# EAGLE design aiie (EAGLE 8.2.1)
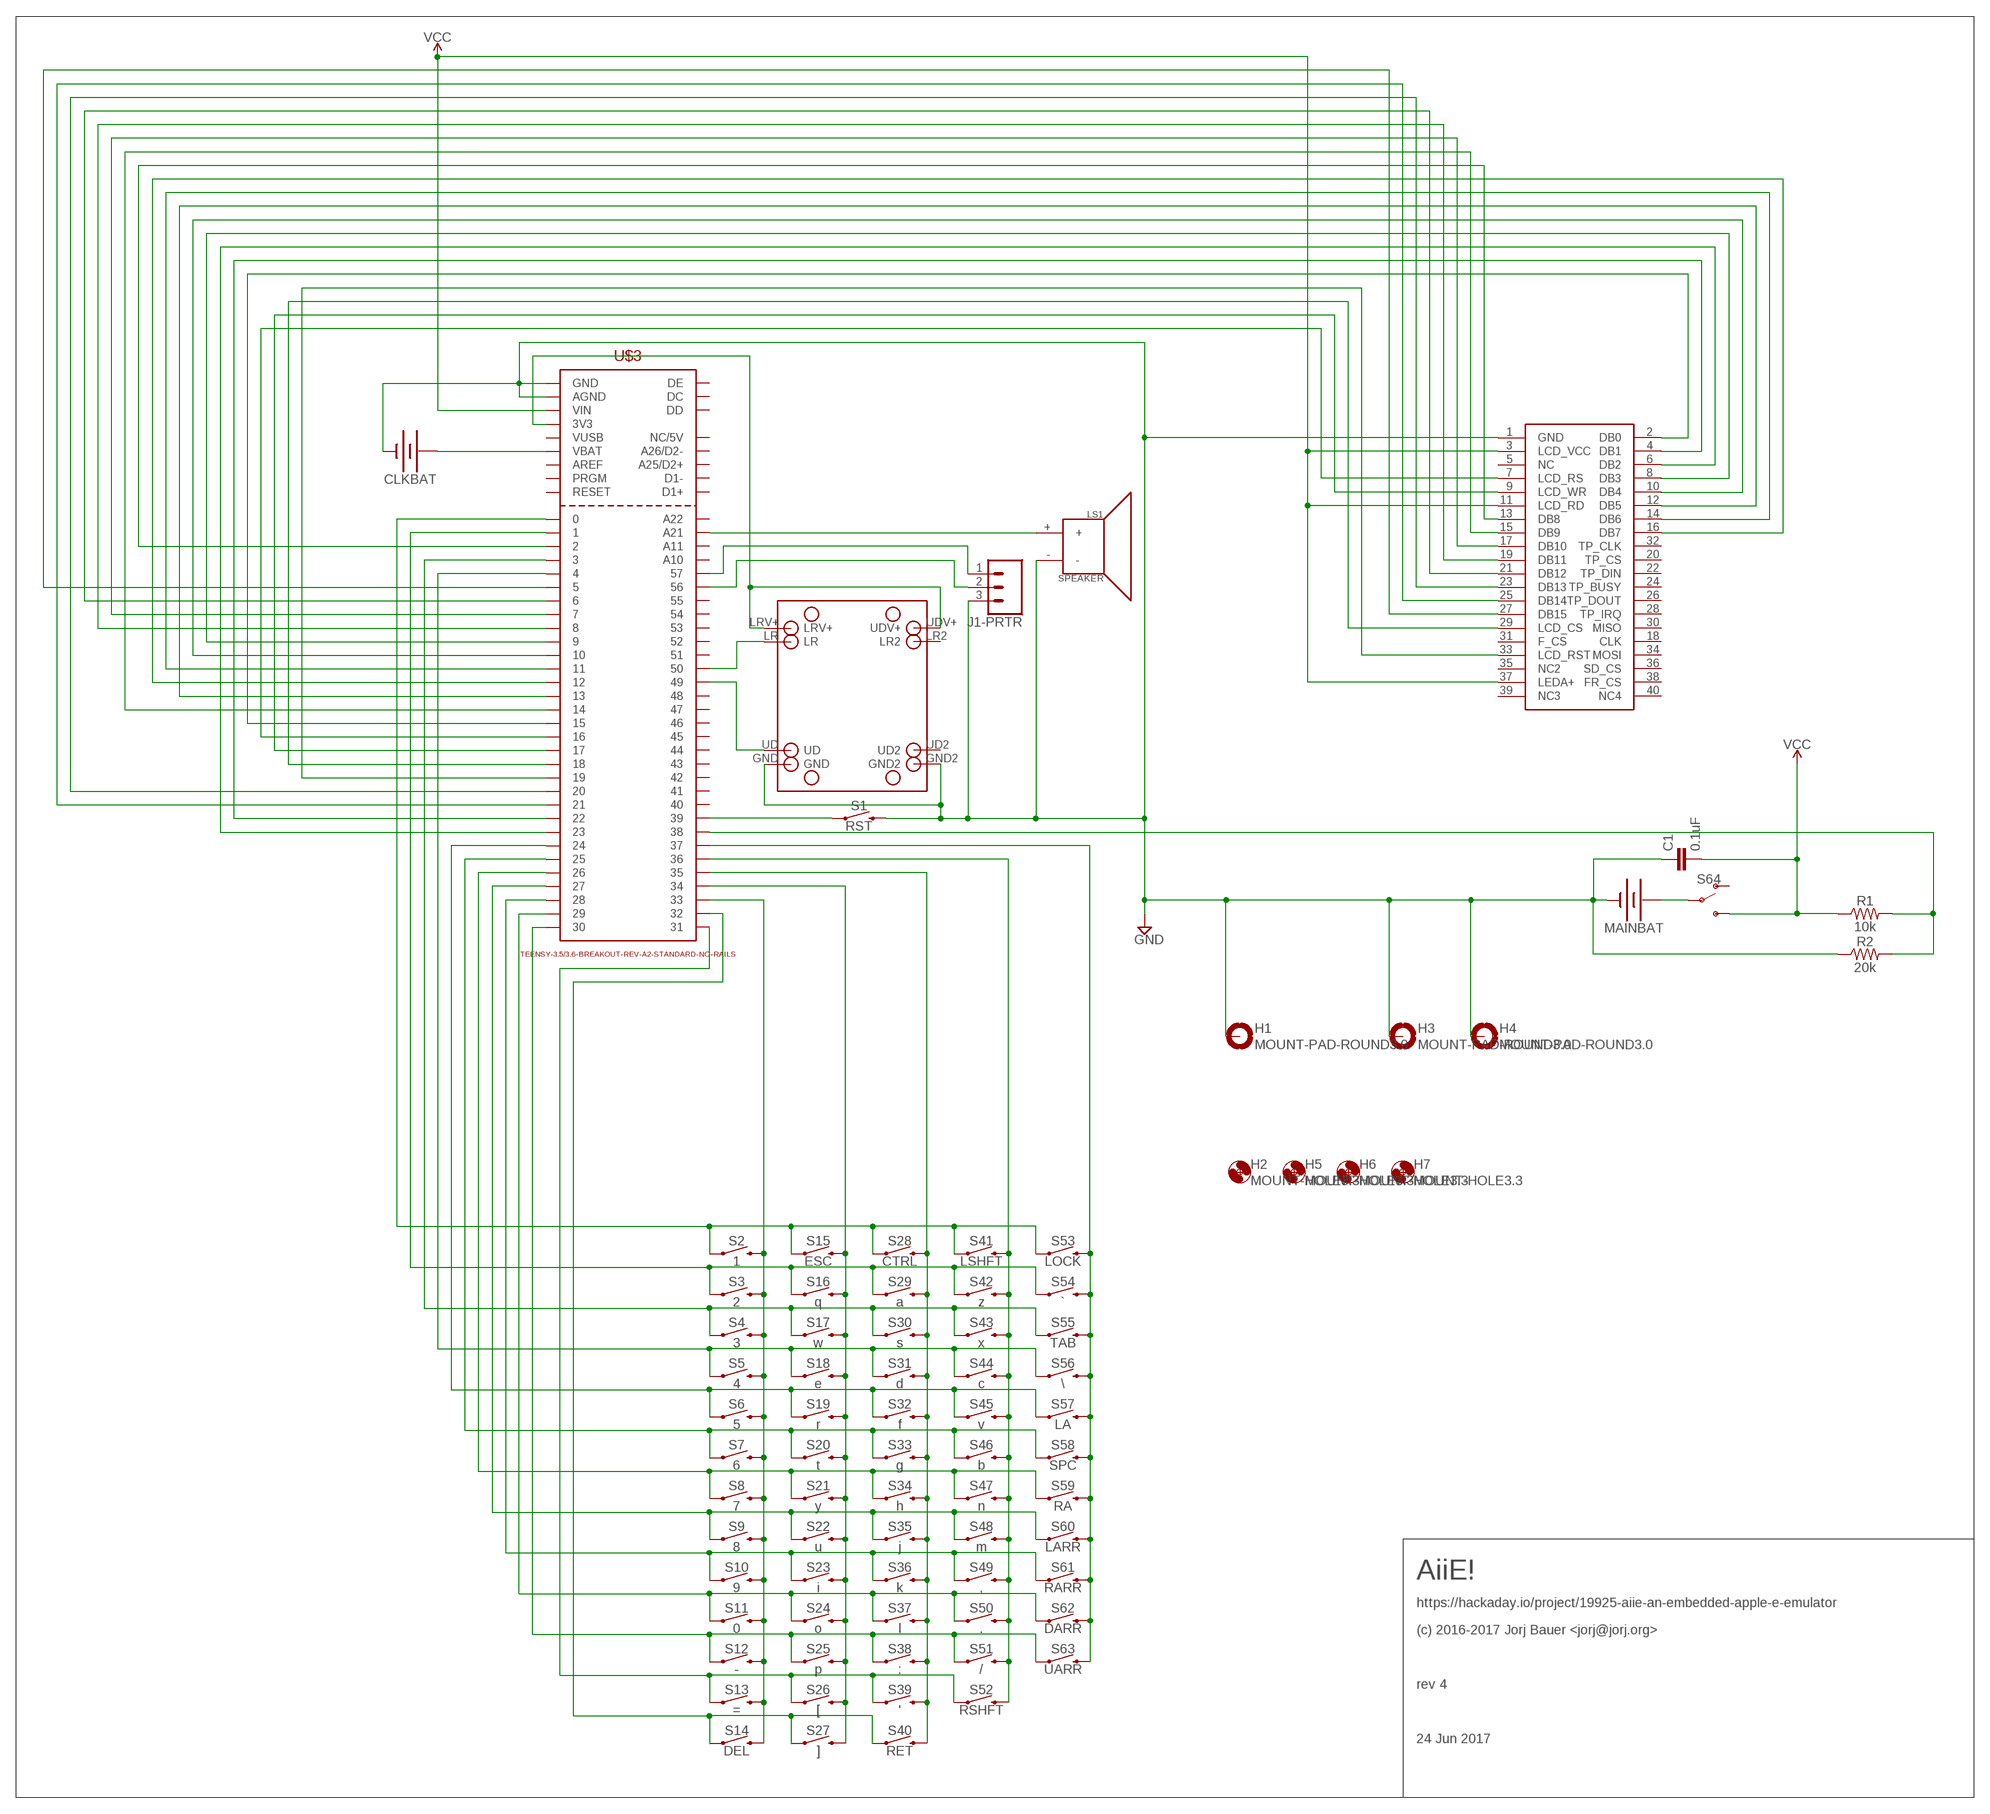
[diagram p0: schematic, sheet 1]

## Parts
C1  0.1uF  C-EU025_050-025X075  [C025_050-025X075]
CLKBAT  BATTERY-20MM_PTH  [BATTCOM_20MM_PTH]
H1  MOUNT-PAD-ROUND3.0  [3,0-PAD]
H2  MOUNT-HOLE3.3  [3,3]
H3  MOUNT-PAD-ROUND3.0  [3,0-PAD]
H4  MOUNT-PAD-ROUND3.0  [3,0-PAD]
H5  MOUNT-HOLE3.3  [3,3]
H6  MOUNT-HOLE3.3  [3,3]
H7  MOUNT-HOLE3.3  [3,3]
J1-PRTR  CONN_03  [1X03]
LS1  SPEAKER  [PCB_MOUNT_SPEAKER]
MAINBAT  BATTERY-18650  [BATTERY_18650-HOLDER]
R1  10k  10KOHM-HORIZ-1/4W-1%  [AXIAL-0.3]
R2  20k  10KOHM-HORIZ-1/4W-1%  [AXIAL-0.3]
S1  RST  MOMENTARY-SWITCH-SPST-PTH-6.0MM  [TACTILE_SWITCH_PTH_6.0MM]
S2  1  MOMENTARY-SWITCH-SPST-PTH-6.0MM  [TACTILE_SWITCH_PTH_6.0MM]
S3  2  MOMENTARY-SWITCH-SPST-PTH-6.0MM  [TACTILE_SWITCH_PTH_6.0MM]
S4  3  MOMENTARY-SWITCH-SPST-PTH-6.0MM  [TACTILE_SWITCH_PTH_6.0MM]
S5  4  MOMENTARY-SWITCH-SPST-PTH-6.0MM  [TACTILE_SWITCH_PTH_6.0MM]
S6  5  MOMENTARY-SWITCH-SPST-PTH-6.0MM  [TACTILE_SWITCH_PTH_6.0MM]
S7  6  MOMENTARY-SWITCH-SPST-PTH-6.0MM  [TACTILE_SWITCH_PTH_6.0MM]
S8  7  MOMENTARY-SWITCH-SPST-PTH-6.0MM  [TACTILE_SWITCH_PTH_6.0MM]
S9  8  MOMENTARY-SWITCH-SPST-PTH-6.0MM  [TACTILE_SWITCH_PTH_6.0MM]
S10  9  MOMENTARY-SWITCH-SPST-PTH-6.0MM  [TACTILE_SWITCH_PTH_6.0MM]
S11  0  MOMENTARY-SWITCH-SPST-PTH-6.0MM  [TACTILE_SWITCH_PTH_6.0MM]
S12  -  MOMENTARY-SWITCH-SPST-PTH-6.0MM  [TACTILE_SWITCH_PTH_6.0MM]
S13  =  MOMENTARY-SWITCH-SPST-PTH-6.0MM  [TACTILE_SWITCH_PTH_6.0MM]
S14  DEL  MOMENTARY-SWITCH-SPST-PTH-6.0MM  [TACTILE_SWITCH_PTH_6.0MM]
S15  ESC  MOMENTARY-SWITCH-SPST-PTH-6.0MM  [TACTILE_SWITCH_PTH_6.0MM]
S16  q  MOMENTARY-SWITCH-SPST-PTH-6.0MM  [TACTILE_SWITCH_PTH_6.0MM]
S17  w  MOMENTARY-SWITCH-SPST-PTH-6.0MM  [TACTILE_SWITCH_PTH_6.0MM]
S18  e  MOMENTARY-SWITCH-SPST-PTH-6.0MM  [TACTILE_SWITCH_PTH_6.0MM]
S19  r  MOMENTARY-SWITCH-SPST-PTH-6.0MM  [TACTILE_SWITCH_PTH_6.0MM]
S20  t  MOMENTARY-SWITCH-SPST-PTH-6.0MM  [TACTILE_SWITCH_PTH_6.0MM]
S21  y  MOMENTARY-SWITCH-SPST-PTH-6.0MM  [TACTILE_SWITCH_PTH_6.0MM]
S22  u  MOMENTARY-SWITCH-SPST-PTH-6.0MM  [TACTILE_SWITCH_PTH_6.0MM]
S23  i  MOMENTARY-SWITCH-SPST-PTH-6.0MM  [TACTILE_SWITCH_PTH_6.0MM]
S24  o  MOMENTARY-SWITCH-SPST-PTH-6.0MM  [TACTILE_SWITCH_PTH_6.0MM]
S25  p  MOMENTARY-SWITCH-SPST-PTH-6.0MM  [TACTILE_SWITCH_PTH_6.0MM]
S26  [  MOMENTARY-SWITCH-SPST-PTH-6.0MM  [TACTILE_SWITCH_PTH_6.0MM]
S27  ]  MOMENTARY-SWITCH-SPST-PTH-6.0MM  [TACTILE_SWITCH_PTH_6.0MM]
S28  CTRL  MOMENTARY-SWITCH-SPST-PTH-6.0MM  [TACTILE_SWITCH_PTH_6.0MM]
S29  a  MOMENTARY-SWITCH-SPST-PTH-6.0MM  [TACTILE_SWITCH_PTH_6.0MM]
S30  s  MOMENTARY-SWITCH-SPST-PTH-6.0MM  [TACTILE_SWITCH_PTH_6.0MM]
S31  d  MOMENTARY-SWITCH-SPST-PTH-6.0MM  [TACTILE_SWITCH_PTH_6.0MM]
S32  f  MOMENTARY-SWITCH-SPST-PTH-6.0MM  [TACTILE_SWITCH_PTH_6.0MM]
S33  g  MOMENTARY-SWITCH-SPST-PTH-6.0MM  [TACTILE_SWITCH_PTH_6.0MM]
S34  h  MOMENTARY-SWITCH-SPST-PTH-6.0MM  [TACTILE_SWITCH_PTH_6.0MM]
S35  j  MOMENTARY-SWITCH-SPST-PTH-6.0MM  [TACTILE_SWITCH_PTH_6.0MM]
S36  k  MOMENTARY-SWITCH-SPST-PTH-6.0MM  [TACTILE_SWITCH_PTH_6.0MM]
S37  l  MOMENTARY-SWITCH-SPST-PTH-6.0MM  [TACTILE_SWITCH_PTH_6.0MM]
S38  ;  MOMENTARY-SWITCH-SPST-PTH-6.0MM  [TACTILE_SWITCH_PTH_6.0MM]
S39  '  MOMENTARY-SWITCH-SPST-PTH-6.0MM  [TACTILE_SWITCH_PTH_6.0MM]
S40  RET  MOMENTARY-SWITCH-SPST-PTH-6.0MM  [TACTILE_SWITCH_PTH_6.0MM]
S41  LSHFT  MOMENTARY-SWITCH-SPST-PTH-6.0MM  [TACTILE_SWITCH_PTH_6.0MM]
S42  z  MOMENTARY-SWITCH-SPST-PTH-6.0MM  [TACTILE_SWITCH_PTH_6.0MM]
S43  x  MOMENTARY-SWITCH-SPST-PTH-6.0MM  [TACTILE_SWITCH_PTH_6.0MM]
S44  c  MOMENTARY-SWITCH-SPST-PTH-6.0MM  [TACTILE_SWITCH_PTH_6.0MM]
S45  v  MOMENTARY-SWITCH-SPST-PTH-6.0MM  [TACTILE_SWITCH_PTH_6.0MM]
S46  b  MOMENTARY-SWITCH-SPST-PTH-6.0MM  [TACTILE_SWITCH_PTH_6.0MM]
S47  n  MOMENTARY-SWITCH-SPST-PTH-6.0MM  [TACTILE_SWITCH_PTH_6.0MM]
S48  m  MOMENTARY-SWITCH-SPST-PTH-6.0MM  [TACTILE_SWITCH_PTH_6.0MM]
S49  ,  MOMENTARY-SWITCH-SPST-PTH-6.0MM  [TACTILE_SWITCH_PTH_6.0MM]
S50  .  MOMENTARY-SWITCH-SPST-PTH-6.0MM  [TACTILE_SWITCH_PTH_6.0MM]
S51  /  MOMENTARY-SWITCH-SPST-PTH-6.0MM  [TACTILE_SWITCH_PTH_6.0MM]
S52  RSHFT  MOMENTARY-SWITCH-SPST-PTH-6.0MM  [TACTILE_SWITCH_PTH_6.0MM]
S53  LOCK  MOMENTARY-SWITCH-SPST-PTH-6.0MM  [TACTILE_SWITCH_PTH_6.0MM]
S54  `  MOMENTARY-SWITCH-SPST-PTH-6.0MM  [TACTILE_SWITCH_PTH_6.0MM]
S55  TAB  MOMENTARY-SWITCH-SPST-PTH-6.0MM  [TACTILE_SWITCH_PTH_6.0MM]
S56  \\  MOMENTARY-SWITCH-SPST-PTH-6.0MM  [TACTILE_SWITCH_PTH_6.0MM]
S57  LA  MOMENTARY-SWITCH-SPST-PTH-6.0MM  [TACTILE_SWITCH_PTH_6.0MM]
S58  SPC  MOMENTARY-SWITCH-SPST-PTH-6.0MM  [TACTILE_SWITCH_PTH_6.0MM]
S59  RA  MOMENTARY-SWITCH-SPST-PTH-6.0MM  [TACTILE_SWITCH_PTH_6.0MM]
S60  LARR  MOMENTARY-SWITCH-SPST-PTH-6.0MM  [TACTILE_SWITCH_PTH_6.0MM]
S61  RARR  MOMENTARY-SWITCH-SPST-PTH-6.0MM  [TACTILE_SWITCH_PTH_6.0MM]
S62  DARR  MOMENTARY-SWITCH-SPST-PTH-6.0MM  [TACTILE_SWITCH_PTH_6.0MM]
S63  UARR  MOMENTARY-SWITCH-SPST-PTH-6.0MM  [TACTILE_SWITCH_PTH_6.0MM]
S64  SWITCH-SPDT-PTH-11.6X4.0MM  [SWITCH_SPDT_PTH_11.6X4.0MM]
U$1  PARALLAX2AXIS  [PARALLAX2AXIS]
U$2  SAINSMART32LCDRAW  [2X20]
U$3  TEENSY-3.5/3.6-BREAKOUT-REV-A2-STANDARD-NO-RAILS  [TEENSY-3.5/3.6-BREAKOUT-REV-A2-STANDARD-NO-RAILS]

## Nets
GND [ground]: C1.1 CLKBAT.2(-) H1.B3,0(MOUNT) H3.B3,0(MOUNT) H4.B3,0(MOUNT) J1-PRTR.3 LS1.- MAINBAT.GND@1(-) R2.P$1 S1.3 U$1.GND U$1.GND2 U$2.1(GND) U$3.AGND U$3.GND@1(GND) U$3.GND@2(GND)
N$1: S1.1 U$3.39
N$2: S2.3 S3.3 S4.3 S5.3 S6.3 S7.3 S8.3 S9.3 S10.3 S11.3 S12.3 S13.3 S14.3 U$3.33
N$3: S15.3 S16.3 S17.3 S18.3 S19.3 S20.3 S21.3 S22.3 S23.3 S24.3 S25.3 S26.3 S27.3 U$3.34
N$4: S28.3 S29.3 S30.3 S31.3 S32.3 S33.3 S34.3 S35.3 S36.3 S37.3 S38.3 S39.3 S40.3 U$3.35
N$5: S41.3 S42.3 S43.3 S44.3 S45.3 S46.3 S47.3 S48.3 S49.3 S50.3 S51.3 S52.3 U$3.36
N$6: S53.3 S54.3 S55.3 S56.3 S57.3 S58.3 S59.3 S60.3 S61.3 S62.3 S63.3 U$3.37
N$7: S2.1 S15.1 S28.1 S41.1 S53.1 U$3.0
N$8: S4.1 S17.1 S30.1 S43.1 S55.1 U$3.3
N$9: S3.1 S16.1 S29.1 S42.1 S54.1 U$3.1
N$10: U$2.7(LCD_RS) U$3.16
N$11: S5.1 S18.1 S31.1 S44.1 S56.1 U$3.4
N$12: U$2.9(LCD_WR) U$3.17
N$13: S6.1 S19.1 S32.1 S45.1 S57.1 U$3.24
N$14: U$2.29(LCD_CS) U$3.18
N$15: S7.1 S20.1 S33.1 S46.1 S58.1 U$3.25
N$16: U$2.33(LCD_RST) U$3.19
N$17: S8.1 S21.1 S34.1 S47.1 S59.1 U$3.26
N$18: U$2.2(DB0) U$3.15
N$19: S9.1 S22.1 S35.1 S48.1 S60.1 U$3.27
N$20: U$2.4(DB1) U$3.22
N$21: S10.1 S23.1 S36.1 S49.1 S61.1 U$3.28
N$22: U$2.6(DB2) U$3.23
N$23: S11.1 S24.1 S37.1 S50.1 S62.1 U$3.29
N$24: U$2.8(DB3) U$3.9
N$25: S12.1 S25.1 S38.1 S51.1 S63.1 U$3.30
N$26: S13.1 S26.1 S39.1 S52.1 U$3.31
N$27: S14.1 S27.1 S40.1 U$3.32
N$28: U$2.10(DB4) U$3.10
N$29: U$2.12(DB5) U$3.13
N$30: U$2.14(DB6) U$3.11
N$31: U$2.16(DB7) U$3.12
N$32: U$2.13(DB8) U$3.2
N$33: U$2.15(DB9) U$3.14
N$34: U$2.17(DB10) U$3.7
N$35: U$2.19(DB11) U$3.8
N$36: U$2.21(DB12) U$3.6
N$37: U$2.23(DB13) U$3.20
N$38: U$2.25(DB14) U$3.21
N$39: U$2.27(DB15) U$3.5
N$40 [vcc]: MAINBAT.PWR@1(+) S64.2(P)
N$41: LS1.+ U$3.A21
N$42: U$1.LR U$3.50
N$43: J1-PRTR.2 U$3.56
N$44: R1.P$2 R2.P$2 U$3.38
N$45: J1-PRTR.1 U$3.57
N$46: U$1.UD U$3.49
N$47: U$1.LRV+ U$1.UDV+ U$3.3V3
N$48: CLKBAT.1(+) U$3.VBAT
VCC [vcc]: C1.2 R1.P$1 S64.3(S) U$2.3(LCD_VCC) U$2.11(LCD_RD) U$2.37(LEDA+) U$3.VIN
Unconnected: S64.1(O) U$1.LR2 U$1.UD2 U$2.5(NC) U$2.18(CLK) U$2.20(TP_CS) U$2.22(TP_DIN) U$2.24(TP_BUSY) U$2.26(TP_DOUT) U$2.28(TP_IRQ) U$2.30(MISO) U$2.31(F_CS) U$2.32(TP_CLK) U$2.34(MOSI) U$2.35(NC2) U$2.36(SD_CS) U$2.38(FR_CS) U$2.39(NC3) U$2.40(NC4) U$3.40 U$3.41 U$3.42 U$3.43 U$3.44 U$3.45 U$3.46 U$3.47 U$3.48 U$3.51 U$3.52 U$3.53 U$3.54 U$3.55 U$3.A10 U$3.A11 U$3.A22 U$3.A25/D2+ U$3.A26/D2- U$3.AREF U$3.D1+ U$3.D1- U$3.DC U$3.DD U$3.DE U$3.NC/V5(NC/5V) U$3.PRGM U$3.RESET U$3.VUSB

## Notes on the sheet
- AiiE!
- https://hackaday.io/project/19925-aiie-an-embedded-apple-e-emulator
- (c) 2016-2017 Jorj Bauer <jorj@jorj.org>
- rev 4
- 24 Jun 2017

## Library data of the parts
C1 = rcl:C-EU: CAPACITOR, European symbol
CLKBAT = SparkFun-Batteries:BATTERY: Battery - Single Cell; PROD_ID: BATT-09031; SF_SKU: PRT-00783
H1 H3 H4 = holes:MOUNT-PAD-ROUND: MOUNTING PAD, round
H2 H5-H7 = holes:MOUNT-HOLE: MOUNTING HOLE with drill center marker
J1-PRTR = SparkFun-Connectors:CONN_03: Multi connection point. Often used as Generic Header-pin footprint for 0.1 inch spaced/style header connections On any of the 0.1 inch spaced packages, you can populate with these: Break Away Headers - Straight (PRT-00116) Break Away Male Headers - Right Angle (PRT-00553) Female Headers (PRT-00115)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
LS1 = SparkFun-Electromechanical:SPEAKER: Speaker; PROD_ID: COMP-11789; SF_SKU: COM-11089
MAINBAT = SparkFun-Batteries:BATTERY: Battery - Single Cell; PROD_ID: BATT-12327; SF_SKU: PRT-13113
R1 = SparkFun-Resistors:10KOHM: 10kΩ resistor; PROD_ID: RES-12183
R2 = SparkFun-Resistors:10KOHM: 10kΩ resistor; PROD_ID: RES-12183; VALUE: 10k
S1-S63 = SparkFun-Switches:MOMENTARY-SWITCH-SPST: Momentary Switch (Pushbutton) - SPST; PROD_ID: SWCH-08441; SF_SKU: COM-00097
S64 = SparkFun-Switches:SWITCH-SPDT: Single Pole, Double Throw (SPDT) Switch Single-pole, double-throw (SPDT) switch. Variant Overview SMD-AYZ0202 Surface Mount DPDT Switch (COM-00597) Used on e.g. LilyPad Arduino USB - ATmega32U4 Board PTH-11.6X4.0MM SPDT Mini Power Switch (COM-00102) Used on e.g. SparkFun Simon Says - Through-Hole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; PROD_ID: SWCH-08261; SF_SKU: COM-00102
U$1 = jorjlib:PARALLAX2AXIS
U$2 = jorjlib:SAINSMART32LCD
U$3 = Teensy-Breakout-Eagle-Library:TEENSY-3.5/3.6-BREAKOUT-REV-A2-STANDARD

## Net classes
0 default: width 0.254 mm, clearance 0.203 mm
1 ground: width 0.356 mm, clearance 0.203 mm
2 vcc: width 0.356 mm, clearance 0.203 mm

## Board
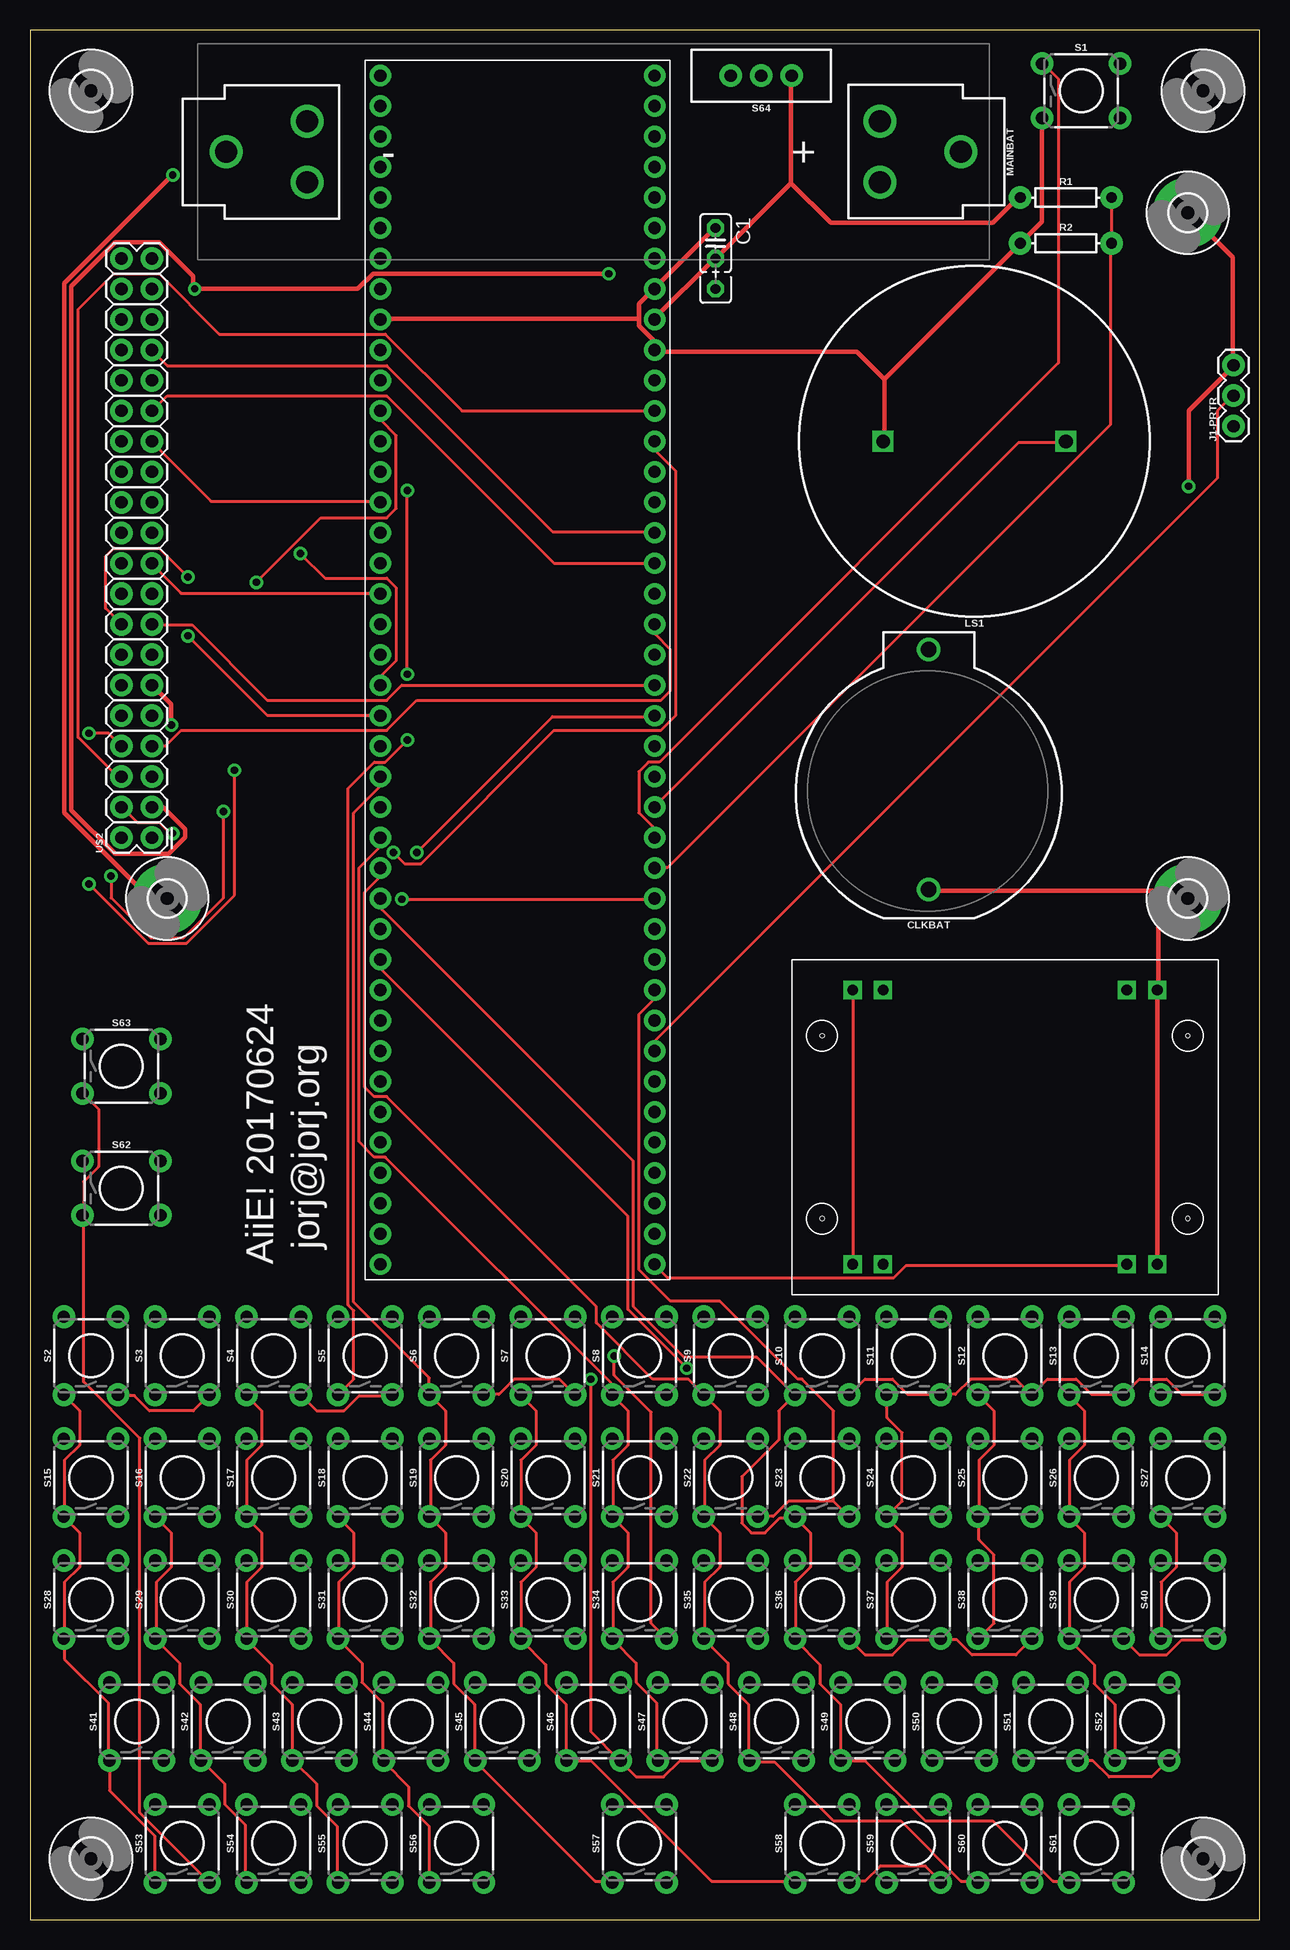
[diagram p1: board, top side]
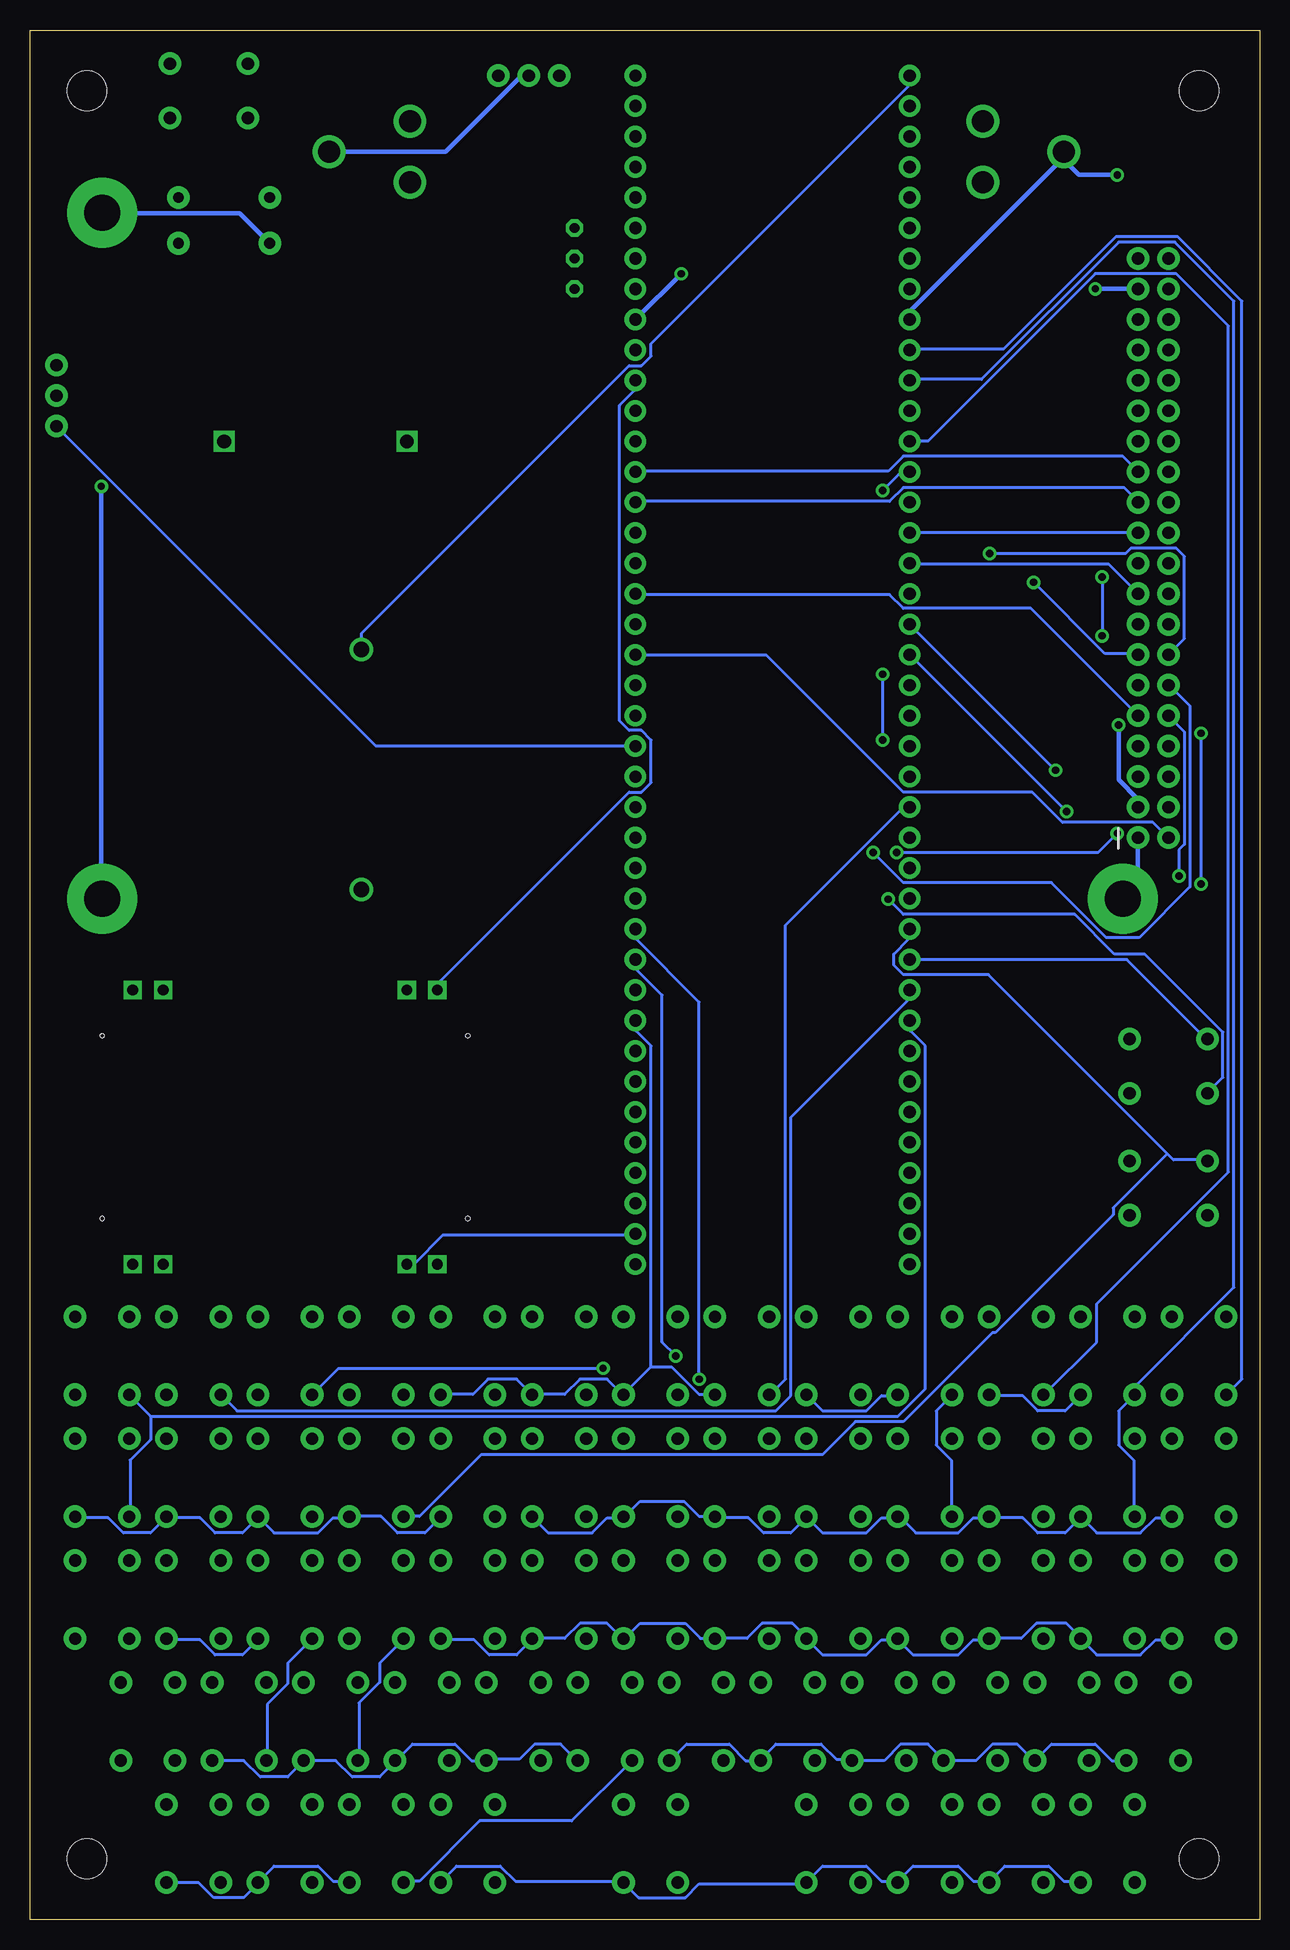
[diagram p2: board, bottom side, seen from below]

Size 102.54 x 157.47 mm. Coordinates in mm from the lower left corner, seen from the top.
Outline: 0,0 102.54,0 102.54,157.47 0,157.47 0,0
Copper layers (1*16): Top 0.035mm / dielectric 1.5mm / Bottom 0.035mm
Design rules "default *": minimum track width 10mil, minimum drill 24mil, track to track 8mil, track to pad 8mil, pad to pad 8mil, via to via 8mil, smd to smd 8mil, copper to edge 40mil, drill to drill 8mil, minimum pad ring 12mil, minimum via ring 10mil, stop-mask expansion 4mil, vias tented up to drill 0mil, thermal gap 10mil

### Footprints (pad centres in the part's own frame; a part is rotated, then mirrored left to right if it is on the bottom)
C025_050-025X075 = drill 0.813 octagon: 1 -1.27,0; 2 1.27,0; 3 3.81,0
BATTCOM_20MM_PTH = drill 1.3: 1 11.85,0; 2 -8.15,0
3,0-PAD = drill 3 pad 5.842: B3,0 0,0
3,3 = hole 3.3: 0,0
1X03 = drill 1.016 pad 1.88: 1 0,0; 2 2.54,0; 3 5.08,0
PCB_MOUNT_SPEAKER = drill 1.143 square: + -7.62,0; - 7.62,0
BATTERY_18650-HOLDER = drill 1.829: GND@1 30.628,0.01; GND@2 23.88,2.55; GND@3 23.88,-2.53; PWR@1 -30.628,-0.01; PWR@2 -23.88,2.53; PWR@3 -23.88,-2.55
AXIAL-0.3 = drill 0.9 pad 1.88: P$1 -3.81,0; P$2 3.81,0
TACTILE_SWITCH_PTH_6.0MM = drill 1.016 pad 1.88: 1 -3.251,2.261; 2 3.251,2.261; 3 -3.251,-2.261; 4 3.251,-2.261
SWITCH_SPDT_PTH_11.6X4.0MM = drill 1.016 pad 1.88: 1 0,2.54; 2 0,0; 3 0,-2.54
PARALLAX2AXIS = drill 0.9 square: GND 2.54,5.08; GND2 25.4,5.08; LR 2.54,27.94; LR2 25.4,27.94; LRV+ 2.54,30.48; UD 2.54,7.62; UD2 25.4,7.62; UDV+ 25.4,30.48 | hole 0.35: 21.59,33.02; 6.35,33.02; 6.35,2.54; 21.59,2.54
2X20 = drill 1.016 pad 1.88: 1 0,0; 2 0,2.54; 3 2.54,0; 4 2.54,2.54; 5 5.08,0; 6 5.08,2.54; 7 7.62,0; 8 7.62,2.54; 9 10.16,0; 10 10.16,2.54; 11 12.7,0; 12 12.7,2.54; 13 15.24,0; 14 15.24,2.54; 15 17.78,0; 16 17.78,2.54; 17 20.32,0; 18 20.32,2.54; 19 22.86,0; 20 22.86,2.54; 21 25.4,0; 22 25.4,2.54; 23 27.94,0; 24 27.94,2.54; 25 30.48,0; 26 30.48,2.54; 27 33.02,0; 28 33.02,2.54; 29 35.56,0; 30 35.56,2.54; 31 38.1,0; 32 38.1,2.54; 33 40.64,0; 34 40.64,2.54; 35 43.18,0; 36 43.18,2.54; 37 45.72,0; 38 45.72,2.54; 39 48.26,0; 40 48.26,2.54
TEENSY-3.5/3.6-BREAKOUT-REV-A2-STANDARD-NO-RAILS = drill 1.016 pad 1.778: 0 24.13,1.27; 1 26.67,1.27; 2 29.21,1.27; 3 31.75,1.27; 3V3 26.67,24.13; 4 34.29,1.27; 5 36.83,1.27; 6 39.37,1.27; 7 41.91,1.27; 8 44.45,1.27; 9 46.99,1.27; 10 49.53,1.27; 11 52.07,1.27; 12 54.61,1.27; 13 54.61,24.13; 14 52.07,24.13; 15 49.53,24.13; 16 46.99,24.13; 17 44.45,24.13; 18 41.91,24.13; 19 39.37,24.13; 20 36.83,24.13; 21 34.29,24.13; 22 31.75,24.13; 23 29.21,24.13; 24 59.69,1.27; 25 62.23,1.27; 26 64.77,1.27; 27 67.31,1.27; 28 69.85,1.27; 29 72.39,1.27; 30 74.93,1.27; 31 77.47,1.27; 32 80.01,1.27; 33 80.01,24.13; 34 77.47,24.13; 35 74.93,24.13; 36 72.39,24.13; 37 69.85,24.13; 38 67.31,24.13; 39 64.77,24.13; 40 57.15,1.27; 41 82.55,1.27; 42 85.09,1.27; 43 87.63,1.27; 44 90.17,1.27; 45 92.71,1.27; 46 95.25,1.27; 47 97.79,1.27; 48 100.33,1.27; 49 100.33,24.13; 50 97.79,24.13; 51 95.25,24.13; 52 92.71,24.13; 53 90.17,24.13; 54 87.63,24.13; 55 85.09,24.13; 56 82.55,24.13; 57 57.15,24.13; A10 16.51,1.27; A11 19.05,1.27; A21 62.23,24.13; A22 59.69,24.13; A25/D2+ 8.89,1.27; A26/D2- 6.35,1.27; AGND 24.13,24.13; AREF 8.89,24.13; D1+ 13.97,1.27; D1- 11.43,1.27; DC 3.81,24.13; DD 1.27,24.13; DE 6.35,24.13; GND@1 21.59,1.27; GND@2 19.05,24.13; NC/V5 3.81,1.27; PRGM 13.97,24.13; RESET 11.43,24.13; VBAT 1.27,1.27; VIN 21.59,24.13; VUSB 16.51,24.13

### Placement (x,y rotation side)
C1  57.15,139.7 270 top
CLKBAT  74.93,93.98 90 top
H1  11.43,85.09 0 top
H2  97.79,5.08 0 top
H3  96.52,142.24 0 top
H4  96.52,85.09 0 top
H5  5.08,5.08 0 top
H6  97.79,152.4 0 top
H7  5.08,152.4 0 top
J1-PRTR  100.33,124.46 90 top
LS1  78.74,123.19 180 top
MAINBAT  46.99,147.32 180 top
R1  86.36,143.51 0 top
R2  86.36,139.7 0 top
S1  87.63,152.4 0 top
S2  5.08,46.99 90 top
S3  12.7,46.99 90 top
S4  20.32,46.99 90 top
S5  27.94,46.99 90 top
S6  35.56,46.99 90 top
S7  43.18,46.99 90 top
S8  50.8,46.99 90 top
S9  58.42,46.99 90 top
S10  66.04,46.99 90 top
S11  73.66,46.99 90 top
S12  81.28,46.99 90 top
S13  88.9,46.99 90 top
S14  96.52,46.99 90 top
S15  5.08,36.83 90 top
S16  12.7,36.83 90 top
S17  20.32,36.83 90 top
S18  27.94,36.83 90 top
S19  35.56,36.83 90 top
S20  43.18,36.83 90 top
S21  50.8,36.83 90 top
S22  58.42,36.83 90 top
S23  66.04,36.83 90 top
S24  73.66,36.83 90 top
S25  81.28,36.83 90 top
S26  88.9,36.83 90 top
S27  96.52,36.83 90 top
S28  5.08,26.67 90 top
S29  12.7,26.67 90 top
S30  20.32,26.67 90 top
S31  27.94,26.67 90 top
S32  35.56,26.67 90 top
S33  43.18,26.67 90 top
S34  50.8,26.67 90 top
S35  58.42,26.67 90 top
S36  66.04,26.67 90 top
S37  73.66,26.67 90 top
S38  81.28,26.67 90 top
S39  88.9,26.67 90 top
S40  96.52,26.67 90 top
S41  8.89,16.51 90 top
S42  16.51,16.51 90 top
S43  24.13,16.51 90 top
S44  31.75,16.51 90 top
S45  39.37,16.51 90 top
S46  46.99,16.51 90 top
S47  54.61,16.51 90 top
S48  62.23,16.51 90 top
S49  69.85,16.51 90 top
S50  77.47,16.51 90 top
S51  85.09,16.51 90 top
S52  92.71,16.51 90 top
S53  12.7,6.35 90 top
S54  20.32,6.35 90 top
S55  27.94,6.35 90 top
S56  35.56,6.35 90 top
S57  50.8,6.35 90 top
S58  66.04,6.35 90 top
S59  73.66,6.35 90 top
S60  81.28,6.35 90 top
S61  88.9,6.35 90 top
S62  7.62,60.96 0 top
S63  7.62,71.12 0 top
S64  60.96,153.67 90 top
U$1  99.06,52.07 90 top
U$2  10.16,90.17 90 top
U$3  27.94,154.94 270 top

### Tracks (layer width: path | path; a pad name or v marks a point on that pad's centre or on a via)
GND  (via drill 0.61)
  Top 0.356: v11.9,145.39 2.87,136.36 2.87,92.24 9.96,85.15 11.33,85.15 H1.B3,0 | U$1.GND 93.97,54.63 93.97,77.38 U$1.GND2 94.08,77.61 94.08,85.61 H4.B3,0 96.48,85.15 95.91,85.72 74.99,85.72 CLKBAT.2 | H3.B3,0 96.6,142.19 100.25,138.53 100.25,129.62 J1-PRTR.3 100.25,129.39 96.6,125.73 v96.6,119.44 | C1.1 57.05,140.93 52.02,135.9 U$3.GND@2 51.91,135.79 50.76,134.65 50.76,133.39 | 50.76,133.39 50.76,132.82 52.02,131.56 52.02,130.87 U$3.AGND 52.13,130.65 68.94,130.65 71.22,128.36 | 71.22,128.36 71.22,123.22 LS1.- | 71.22,128.36 82.54,139.68 R2.P$1 82.65,139.79 84.37,141.5 84.37,150.08 S1.3 | 50.76,133.39 29.27,133.39 U$3.GND@1
  Bottom 0.356: U$2.1 10.18,90.07 10.18,86.3 11.33,85.15 H1.B3,0 | U$3.GND@1 29.16,133.39 29.16,134.07 16.47,146.76 16.47,147.22 MAINBAT.GND@1 16.36,146.65 15.1,145.39 v11.9,145.39 | H3.B3,0 96.48,142.19 85.05,142.19 82.65,139.79 R2.P$1 | v96.6,119.44 96.6,85.15 H4.B3,0
N$1
  Top 0.254: U$3.39 52.02,90.18 52.02,90.98 50.76,92.24 50.76,95.67 51.56,96.47 52.48,96.47 85.74,129.73 85.74,153.39 84.48,154.65 S1.1
N$2
  Top 0.254: S2.3 7.44,43.66 8.7,43.66 9.96,42.41 13.61,42.41 14.87,43.66 S3.3 | S5.3 30.19,43.66 27.45,43.66 26.19,42.41 23.9,42.41 22.64,43.66 S4.3 | S14.3 98.77,43.78 96.02,43.78 94.77,45.03 92.48,45.03 91.22,43.78 S13.3 91.11,43.78 88.48,43.78 87.22,45.03 84.82,45.03 83.57,43.78 S12.3 83.45,43.78 82.19,45.03 78.42,45.03 77.16,43.78 76.02,43.78 S11.3 75.91,43.78 73.16,43.78 71.91,45.03 69.62,45.03 68.36,43.78 S10.3 | S6.3 37.85,43.78 39.1,43.78 40.36,45.03 44.13,45.03 45.39,43.78 S7.3
  Bottom 0.254: S5.3 30.3,43.66 31.56,43.66 32.82,42.41 36.47,42.41 37.73,43.66 S6.3 | S4.3 22.53,43.66 19.79,43.66 18.53,42.41 16.24,42.41 14.99,43.66 S3.3 | 50.76,46.06 50.76,72.81 52.02,74.07 52.02,74.87 U$3.33 | 50.76,46.06 53.05,43.78 S8.3 53.16,43.78 54.42,45.03 56.71,45.03 57.96,43.78 60.59,43.78 S9.3 60.71,43.78 61.96,45.03 64.36,45.03 65.62,43.78 68.25,43.78 S10.3 | 50.76,46.06 49.05,46.06 46.76,43.78 45.5,43.78 S7.3
N$3
  Top 0.254: 66.99,34.86 66.99,42.41 64.36,45.03 64.02,45.03 57.51,51.55 53.39,51.55 50.76,54.18 50.76,75.44 52.02,76.69 52.02,77.38 U$3.34 | 66.99,34.86 68.25,33.6 S23.3 | 66.99,34.86 63.22,34.86 61.96,33.6 60.71,33.6 S22.3
  Bottom 0.254: S15.3 7.44,33.49 8.7,33.49 9.96,32.23 13.61,32.23 S16.3 14.99,33.49 16.24,32.23 18.53,32.23 19.79,33.49 22.53,33.49 S17.3 22.64,33.49 23.9,33.49 25.16,32.23 28.7,32.23 30.07,33.6 S18.3 30.3,33.49 31.56,33.49 32.82,32.23 36.47,32.23 S19.3 37.85,33.49 39.1,32.23 41.39,32.23 42.65,33.49 45.39,33.49 S20.3 45.5,33.6 46.76,33.6 48.02,34.86 51.68,34.86 52.93,33.6 S21.3 53.16,33.49 54.42,33.49 55.68,32.23 59.33,32.23 S22.3 | S27.3 98.77,33.49 96.02,33.49 94.77,32.23 92.48,32.23 91.22,33.49 S26.3 91.11,33.49 88.37,33.49 87.11,32.23 84.82,32.23 83.57,33.49 S25.3 82.19,32.23 78.54,32.23 77.28,33.49 76.02,33.49 S24.3 75.79,33.6 73.28,33.6 71.91,32.23 69.62,32.23 68.36,33.49 S23.3
N$4  (via drill 0.61)
  Top 0.254: S38.3 83.45,23.32 82.19,22.06 78.54,22.06 77.28,23.32 76.02,23.32 S37.3 75.91,23.32 73.16,23.32 71.91,22.06 69.62,22.06 68.36,23.32 S36.3 | S40.3 98.77,23.32 96.02,23.32 94.77,22.06 92.48,22.06 91.22,23.32 S39.3 | v48.7,46.98 48.7,45.38 51.79,42.29 51.79,24.69 S34.3
  Bottom 0.254: S28.3 7.44,23.32 8.7,23.32 9.96,22.06 13.61,22.06 14.87,23.32 S29.3 14.99,23.55 16.13,24.69 18.64,24.69 19.9,23.43 22.53,23.43 S30.3 22.64,23.32 23.9,23.32 25.16,22.06 28.93,22.06 30.19,23.32 S31.3 30.3,23.32 31.56,23.32 32.82,22.06 36.47,22.06 37.73,23.32 S32.3 37.85,23.55 38.99,24.69 41.5,24.69 42.76,23.43 45.39,23.43 S33.3 45.5,23.43 46.65,23.43 47.9,24.69 51.68,24.69 52.93,23.43 S34.3 53.16,23.43 54.42,24.69 56.71,24.69 57.96,23.43 60.59,23.43 S35.3 60.71,23.32 61.96,22.06 64.25,22.06 65.51,23.32 68.25,23.32 S36.3 | S39.3 91.11,23.32 88.37,23.32 87.11,22.06 84.82,22.06 83.57,23.32 S38.3 | v48.7,46.98 49.85,48.12 49.85,77.04 52.02,79.21 52.02,80.01 U$3.35
N$5  (via drill 0.61)
  Top 0.254: S51.3 88.59,13.26 89.97,11.89 93.51,11.89 94.88,13.26 S52.3 | v46.76,45.03 46.76,15.66 49.16,13.26 S46.3 49.28,13.14 50.53,11.89 52.82,11.89 54.19,13.26 S47.3
  Bottom 0.254: S51.3 84.71,13.26 83.34,11.89 81.05,11.89 79.79,13.14 S50.3 77.05,13.26 75.68,11.89 73.39,11.89 72.14,13.14 S49.3 72.02,13.26 70.65,14.63 67.11,14.63 65.73,13.26 S48.3 64.48,13.37 61.74,13.37 60.48,14.63 58.31,14.63 56.93,13.26 S47.3 | S41.3 12.36,13.26 13.73,14.63 17.39,14.63 18.76,13.26 S42.3 18.87,13.26 20.24,14.63 22.3,14.63 23.67,13.26 S43.3 26.42,13.37 27.67,14.63 29.96,14.63 31.33,13.26 S44.3 34.07,13.37 35.33,13.37 36.59,14.63 40.36,14.63 41.62,13.37 S45.3 42.88,13.26 44.25,14.63 47.79,14.63 49.16,13.26 S46.3 | v46.76,45.03 46.76,76.47 52.02,81.72 52.02,82.53 U$3.36
N$6  (via drill 0.61)
  Top 0.254: v30.99,85.04 52.02,85.04 U$3.37 | S63.3 4.47,68.81 5.73,67.55 5.73,62.75 4.47,61.49 4.47,58.75 S62.3 4.47,58.64 4.47,44.81 9.16,40.12 9.16,8.91 14.87,3.2 S53.3 | S58.3 68.36,3.2 69.62,3.2 70.88,4.46 74.65,4.46 75.91,3.2 S59.3
  Bottom 0.254: v30.99,85.04 29.73,83.78 15.44,83.78 12.13,80.47 9.61,80.47 3.1,73.95 3.1,70.18 4.36,68.92 S63.3 | S53.3 14.99,3.2 16.36,3.2 17.61,4.46 21.27,4.46 22.53,3.2 S54.3 22.64,3.2 23.9,3.2 25.16,4.46 28.93,4.46 30.19,3.2 S55.3 30.3,3.2 31.56,3.2 32.82,4.46 36.47,4.46 37.73,3.2 S56.3 37.85,2.97 46.76,2.97 47.9,1.83 51.79,1.83 S57.3 53.16,3.2 62.08,3.2 63.34,4.46 66.99,4.46 68.25,3.2 S58.3 | S59.3 76.02,3.2 77.28,3.2 78.54,4.46 82.19,4.46 83.45,3.2 S60.3 83.57,2.97 84.71,1.83 87.22,1.83 88.48,3.09 91.11,3.09 S61.3
N$7
  Top 0.254: S53.1 10.41,3.2 10.41,6.97 6.64,10.74 6.64,13.14 S41.1 6.53,13.26 6.53,18.06 2.87,21.72 2.87,23.32 S28.1 2.87,23.43 2.87,28.12 4.13,29.38 4.13,32.23 2.87,33.49 S15.1 2.87,33.6 2.87,38.29 4.13,39.55 4.13,42.41 2.87,43.66 S2.1
  Bottom 0.254: U$3.0 29.16,130.87 21.39,130.87 12.01,140.25 6.87,140.25 1.5,134.87 1.5,45.03 2.76,43.78 S2.1
N$8
  Top 0.254: S55.1 25.62,3.2 25.62,7.77 23.9,9.49 23.9,11.32 21.96,13.26 S43.1 21.84,13.37 21.84,17.95 20.13,19.66 20.13,21.26 18.07,23.32 S30.1 18.07,23.43 18.07,28.12 19.33,29.38 19.33,32.23 18.07,33.49 S17.1 18.07,33.6 18.07,38.29 19.33,39.55 19.33,42.41 18.07,43.66 S4.1
  Bottom 0.254: U$3.3 29.16,123.22 27.67,123.22 13.73,137.16 6.98,137.16 2.64,132.82 2.64,62.29 13.61,51.32 13.61,48.12 17.96,43.78 S4.1
N$9
  Top 0.254: S54.1 17.96,3.2 17.96,7.89 16.24,9.6 16.24,11.32 14.3,13.26 S42.1 14.19,13.37 14.19,17.95 12.47,19.66 12.47,21.37 10.53,23.32 S29.1 10.53,23.43 10.53,28.12 11.79,29.38 11.79,32.23 S16.1
  Bottom 0.254: U$3.1 29.16,128.36 23.22,128.36 11.79,139.79 7.1,139.79 2.18,134.87 2.18,52.69 10.41,44.46 10.41,43.78 S3.1 10.53,43.66 11.79,42.41 11.79,39.55 10.53,38.29 10.53,33.6 S16.1
N$10
  Top 0.254: U$3.16 52.13,107.9 52.13,107.1 53.39,105.84 53.39,102.41 52.59,101.61 32.25,101.61 29.73,99.1 12.59,99.1 11.33,97.84 10.18,97.84 U$2.7
N$11  (via drill 0.61)
  Top 0.254: S18.1 25.73,33.49 26.99,32.23 26.99,29.38 25.73,28.12 25.73,23.43 S31.1 25.73,23.32 27.67,21.37 27.67,19.77 29.39,18.06 29.39,13.26 S44.1 29.5,13.14 31.56,11.09 31.56,9.49 33.27,7.77 33.27,3.2 S56.1 | v31.45,103.78 v31.45,119.1 | v31.45,98.3 29.62,96.47 28.7,96.47 26.53,94.3 26.53,51.21 26.99,50.75 26.99,45.03 25.73,43.78 S5.1
  Bottom 0.254: v31.45,119.1 29.96,120.59 29.27,120.59 U$3.4 | v31.45,98.3 v31.45,103.78 | S18.1 25.73,33.6 25.73,38.29 26.99,39.55 26.99,42.41 25.73,43.66 S5.1
N$12
  Bottom 0.254: U$2.9 19.1,109.27 29.73,109.27 30.87,110.41 52.02,110.41 U$3.17
N$13
  Top 0.254: S57.1 48.48,3.2 47.1,3.2 37.16,13.14 S45.1 37.05,13.26 37.05,17.95 35.33,19.66 35.33,21.37 33.39,23.32 S32.1 33.39,23.43 33.39,28.12 34.65,29.38 34.65,32.23 S19.1 33.39,33.6 33.39,38.29 34.65,39.55 34.65,42.41 33.39,43.66 S6.1 33.27,43.78 33.27,45.15 26.99,51.44 26.99,92.24 29.16,94.41 29.16,95.21 U$3.24
N$14
  Top 0.254: U$3.18 52.02,113.04 43.68,113.04 29.73,126.99 11.44,126.99 10.18,125.73 U$2.29
N$15
  Top 0.254: S58.1 63.68,3.2 56.82,3.2 46.76,13.26 S46.1 44.7,13.26 44.7,17.95 42.99,19.66 42.99,21.26 40.93,23.32 S33.1 40.93,23.43 40.93,28.12 42.19,29.38 42.19,32.23 40.93,33.49 S20.1 40.93,33.6 40.93,38.29 42.19,39.55 42.19,42.41 40.93,43.66 S7.1
  Bottom 0.254: U$3.25 29.27,92.7 29.73,92.7 39.56,82.87 39.56,45.03 40.82,43.78 S7.1
N$16
  Top 0.254: U$3.19 52.02,115.67 43.56,115.67 29.73,129.5 11.44,129.5 10.18,130.76 U$2.33
N$17
  Top 0.254: S47.1 52.25,13.26 52.25,18.06 50.53,19.77 50.53,21.37 48.59,23.32 S34.1 48.59,23.43 48.59,28.12 49.85,29.38 49.85,32.23 48.59,33.49 S21.1 48.59,33.6 48.59,38.29 49.85,39.55 49.85,42.41 48.59,43.66 S8.1 48.48,43.78 48.48,44.69 29.62,63.55 28.7,63.55 27.45,64.81 27.45,87.67 29.16,89.38 29.16,90.07 U$3.26
  Bottom 0.254: S59.1 71.34,3.2 70.08,3.2 65.05,8.23 57.39,8.23 52.36,13.26 S47.1
N$18
  Bottom 0.254: U$3.15 52.02,105.39 41.16,105.39 29.73,93.95 18.99,93.95 16.47,91.44 8.93,91.44 7.67,90.18 U$2.2
N$19
  Top 0.254: S60.1 78.99,3.2 77.62,3.2 72.59,8.23 66.99,8.23 62.08,13.14 60.02,13.14 S48.1 59.91,13.26 59.91,17.95 58.19,19.66 58.19,21.37 56.25,23.32 S35.1 56.25,23.43 56.25,28.12 57.51,29.38 57.51,32.23 S22.1 56.25,33.6 56.25,38.29 57.51,39.55 57.51,42.41 56.25,43.66 S9.1 56.13,43.78 54.88,45.03 51.91,45.03 47.22,49.72 47.22,51.09 29.73,68.58 28.7,68.58 27.9,69.38 27.9,85.61 29.16,86.87 29.16,87.55 U$3.27
N$20  (via drill 0.61)
  Top 0.254: v30.3,88.92 31.22,88.01 32.59,88.01 43.68,99.1 52.59,99.1 53.85,100.36 53.85,120.7 52.13,122.42 52.13,123.1 U$3.22 | v11.9,90.53 11.67,90.53 10.76,91.44 8.93,91.44 7.67,92.7 U$2.4
  Bottom 0.254: v30.3,88.92 13.5,88.92 v11.9,90.53
N$21
  Top 0.254: S61.1 86.54,3.2 85.28,3.2 80.25,8.23 74.65,8.23 69.62,13.26 S49.1 67.56,13.26 67.56,17.95 65.85,19.66 65.85,21.26 63.79,23.32 S36.1 63.79,23.43 63.79,28.12 65.05,29.38 65.05,32.23 63.79,33.49 S23.1 63.68,33.49 62.54,33.49 61.28,32.23 60.13,32.23 59.33,33.03 59.33,36.92 62.42,40.01 62.42,42.41 63.68,43.66 S10.1 63.68,43.78 60.59,46.86 54.53,46.86 50.3,51.09 50.3,63.21 29.27,84.24 29.27,85.04 U$3.28
N$22
  Top 0.254: U$3.23 36.02,125.73 29.62,132.13 15.79,132.13 10.76,137.16 6.98,137.16 4.01,134.19 4.01,98.53 7.21,95.33 7.56,95.33 U$2.6
N$23
  Top 0.254: S37.1 71.45,23.43 71.45,28.12 72.71,29.38 72.71,32.23 71.45,33.49 S24.1 71.45,33.6 72.71,34.86 72.71,40.58 71.45,41.83 71.45,43.66 S11.1
  Bottom 0.254: S50.1 75.11,13.26 75.11,18.06 73.39,19.77 73.39,21.37 71.45,23.32 S37.1 | 7.73,63.84 7.21,63.32 4.47,63.32 S62.1 | 7.73,63.84 22.64,78.75 29.73,78.75 30.53,79.55 30.53,80.47 29.27,81.72 29.27,82.53 U$3.29 | 7.73,63.84 12.24,59.32 12.24,58.75 22.07,48.92 22.3,48.92 29.73,41.49 33.73,41.49 36.47,38.75 64.94,38.75 70.08,33.6 71.34,33.6 S24.1
N$24  (via drill 0.61)
  Top 0.254: v17.04,95.78 17.04,85.38 13.04,81.38 9.84,81.38 v4.93,86.3 | v4.93,98.87 6.53,98.87 7.56,97.84 U$2.8
  Bottom 0.254: v17.04,95.78 U$3.9 | v4.93,98.87 v4.93,86.3
N$25  (via drill 0.61)
  Top 0.254: S12.1 79.11,43.66 80.37,42.41 80.37,39.55 79.11,38.29 79.11,33.6 S25.1 79.11,33.49 79.11,31.66 80.37,30.4 80.37,24.69 79.11,23.43 S38.1 | v54.76,45.95 49.85,50.86 49.85,58.64 29.27,79.21 29.27,80.01 U$3.30
  Bottom 0.254: U$3.30 11.1,80.01 4.47,73.38 S63.1 | S51.1 82.77,13.26 82.77,17.95 81.05,19.66 81.05,21.37 79.11,23.32 S38.1 | v54.76,45.95 76.82,45.95 78.99,43.78 S12.1
N$26
  Top 0.254: S52.1 90.42,13.26 90.42,17.95 88.71,19.66 88.71,21.26 86.65,23.32 S39.1 86.65,23.43 86.65,28.12 87.91,29.38 87.91,32.23 86.65,33.49 S26.1 86.65,33.6 86.65,38.29 87.91,39.55 87.91,42.41 86.65,43.66 S13.1
  Bottom 0.254: U$3.31 29.27,77.38 29.27,76.69 39.1,66.86 39.1,43.66 40.36,42.41 85.28,42.41 86.54,43.66 S13.1
N$27
  Top 0.254: S40.1 94.31,23.43 94.31,28.12 95.57,29.38 95.57,32.23 94.31,33.49 S27.1
  Bottom 0.254: 92.48,41.95 30.19,41.95 27.9,44.23 27.9,72.81 29.16,74.07 29.16,74.87 U$3.32 | 92.48,41.95 94.2,43.66 S14.1 | 92.48,41.95 92.48,40.01 94.2,38.29 94.2,33.6 S27.1
N$28  (via drill 0.61)
  Top 0.254: v16.13,92.35 16.13,85.15 12.81,81.84 10.07,81.84 6.76,85.15 v6.76,86.98
  Bottom 0.254: v16.13,92.35 29.16,105.39 U$3.10 | v6.76,86.98 6.76,89.15 6.3,89.61 6.3,98.98 7.56,100.24 U$2.10
N$29  (via drill 0.61)
  Top 0.254: v32.25,88.92 43.56,100.24 52.02,100.24 U$3.13
  Bottom 0.254: v32.25,88.92 29.73,86.41 17.39,86.41 12.81,81.84 10.07,81.84 5.84,86.07 5.84,101.16 7.56,102.87 U$2.12
N$30  (via drill 0.61)
  Top 0.254: v22.53,113.84 24.59,111.78 29.73,111.78 30.53,110.98 30.53,104.93 29.27,103.67 29.27,102.87 U$3.11
  Bottom 0.254: v22.53,113.84 11.21,113.84 10.76,114.3 6.98,114.3 6.3,113.61 6.3,106.76 7.56,105.5 U$2.14
N$31  (via drill 0.61)
  Top 0.254: v13.16,106.98 19.79,100.36 29.16,100.36 U$3.12 | v13.16,111.9 10.76,114.3 6.98,114.3 6.3,113.61 6.3,109.27 U$2.16
  Bottom 0.254: v13.16,111.9 v13.16,106.98
N$32  (via drill 0.61)
  Top 0.254: v18.87,111.44 24.24,116.81 29.73,116.81 30.53,117.61 30.53,123.67 29.27,124.93 29.27,125.73 U$3.2
  Bottom 0.254: v18.87,111.44 12.93,105.5 10.18,105.5 U$2.13
N$33
  Top 0.254: U$3.14 30.99,102.87 29.73,101.61 19.79,101.61 13.5,107.9 10.18,107.9 U$2.15
N$34
  Bottom 0.254: U$3.7 29.16,112.93 12.59,112.93 10.18,110.53 U$2.17
N$35
  Top 0.254: U$3.8 29.16,110.53 12.59,110.53 10.18,112.93 U$2.19
N$36
  Bottom 0.254: U$3.6 29.16,115.56 10.18,115.56 U$2.21
N$37
  Bottom 0.254: U$3.20 52.02,118.19 30.87,118.19 29.73,119.33 11.33,119.33 10.18,118.19 U$2.23
N$38
  Bottom 0.254: U$3.21 52.02,120.7 30.99,120.7 29.73,121.96 11.44,121.96 10.18,120.7 U$2.25
N$39
  Top 0.254: U$3.5 29.16,118.19 15.1,118.19 10.18,123.1 U$2.27
N$40
  Bottom 0.356: S64.2 61.05,153.62 61.62,153.62 67.91,147.33 77.51,147.33 MAINBAT.PWR@1
N$41
  Top 0.254: LS1.+ 86.31,123.1 82.42,123.1 52.13,92.81 U$3.A21
N$42
  Bottom 0.254: U$1.LR 71.11,54.63 70.54,54.63 68.13,57.04 52.25,57.04 52.13,57.15 U$3.50
N$43
  Top 0.254: U$3.56 52.13,72.47 52.13,73.27 99,120.13 99,125.73 100.25,126.99 J1-PRTR.2
N$44
  Top 0.254: U$3.38 52.13,87.67 53.16,87.67 90.08,124.59 90.08,139.68 R2.P$2 90.19,139.79 90.19,143.45 R1.P$2
N$45
  Bottom 0.254: U$3.57 52.13,97.84 73.74,97.84 100.25,124.36 J1-PRTR.1
N$46
  Top 0.254: U$1.UD 91.34,54.52 73.05,54.52 72.02,53.49 53.16,53.49 52.13,54.52 U$3.49
N$47
  Top 0.254: U$1.LRV+ 68.59,54.63 68.59,77.38 U$1.UDV+
  Bottom 0.254: U$3.3V3 52.13,128.25 52.13,127.44 53.39,126.19 53.39,99.9 52.59,99.1 51.56,99.1 50.76,98.3 50.76,94.75 51.56,93.95 52.59,93.95 68.48,78.07 68.48,77.5 U$1.UDV+
N$48
  Bottom 0.254: U$3.VBAT 29.27,153.62 29.27,152.82 50.76,131.33 50.76,130.3 51.56,129.5 52.59,129.5 74.88,107.21 74.88,105.84 CLKBAT.1
VCC  (via drill 0.61)
  Top 0.356: v11.79,99.56 11.79,101.27 10.18,102.87 U$2.11 | U$3.VIN 52.02,133.39 57.05,138.42 C1.2 57.28,138.53 63.45,144.7 | v48.25,137.16 28.59,137.16 27.33,135.9 v13.73,135.9 13.61,136.02 13.61,136.93 10.76,139.79 7.1,139.79 3.44,136.13 3.44,92.47 7.1,88.81 11.56,88.81 12.93,90.18 12.93,90.87 11.1,92.7 10.18,92.7 U$2.3 | 63.45,144.7 63.45,153.62 S64.3 | 63.45,144.7 66.76,141.39 80.25,141.39 82.31,143.45 82.54,143.45 R1.P$1
  Bottom 0.356: v11.79,99.56 11.79,94.98 10.18,93.38 10.18,92.81 U$2.3 | v13.73,135.9 10.18,135.9 U$2.37 | v48.25,137.16 52.02,133.39 U$3.VIN

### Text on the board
tPlace: jorj@jorj.org | AiiE! 20170624

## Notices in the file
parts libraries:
SparkFun-Switches: Licensing: Creative Commons ShareAlike 4.0 International - https://creativecommons.org/licenses/by-sa/4.0
